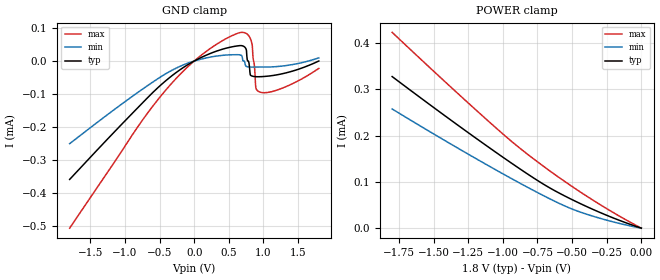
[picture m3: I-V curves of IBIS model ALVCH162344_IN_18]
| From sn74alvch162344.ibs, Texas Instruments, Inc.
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[Model]   ALVCH162344_IN_18
Model_type  Input
Vinl = 0.5775
Vinh = 1.2675
| variable   typ   min   max
C_comp   2.00pF   1.77pF   2.25pF
[Temperature Range]   40   100   -40
| Ambient temperature   25   85   -40
[Voltage range]   1.8   1.65   1.95
[GND Clamp]
| ALVCH162344_IN_18
|   Voltage   I(typ)   I(min)   I(max)
-1.8V     -358.2uA   -250uA     -505.6uA
-525mV    -80.66uA   -53.43uA   -116.9uA
320mV     29.78uA    14.92uA    50.35uA
700mV     45.75uA    3.679uA    86.65uA
750mV     35.67uA    -15.88uA   83.67uA
780mV     -24.55nA   -17.79uA   78.47uA
810mV     -41.75uA   -18.34uA   68.19uA
840mV     -45.74uA   -18.35uA   44.73uA
870mV     -46.96uA   -18.34uA   -15.03uA
890mV     -47.36uA   -18.33uA   -80.84uA
960mV     -47.37uA   -18.3uA    -94.73uA
1.8V      4.586pA    9.591uA    -22.36uA
[POWER Clamp]
| ALVCH162344_IN_18
|   Voltage   I(typ)   I(min)   I(max)
-1.8V     327.9uA    257.8uA    423.5uA
-1.395V   237.9uA    185.2uA    310.4uA
-1.055V   164.9uA    126.7uA    218.2uA
-890mV    130.8uA    99.39uA    176uA
-705mV    94.78uA    70.07uA    133.4uA
-545mV    68.39uA    47.01uA    99.32uA
-410mV    48.8uA     31.61uA    72.23uA
-205mV    22.33uA    13.68uA    34.16uA
-16.28fV  4.586pA    5.339pA    4.458pA
